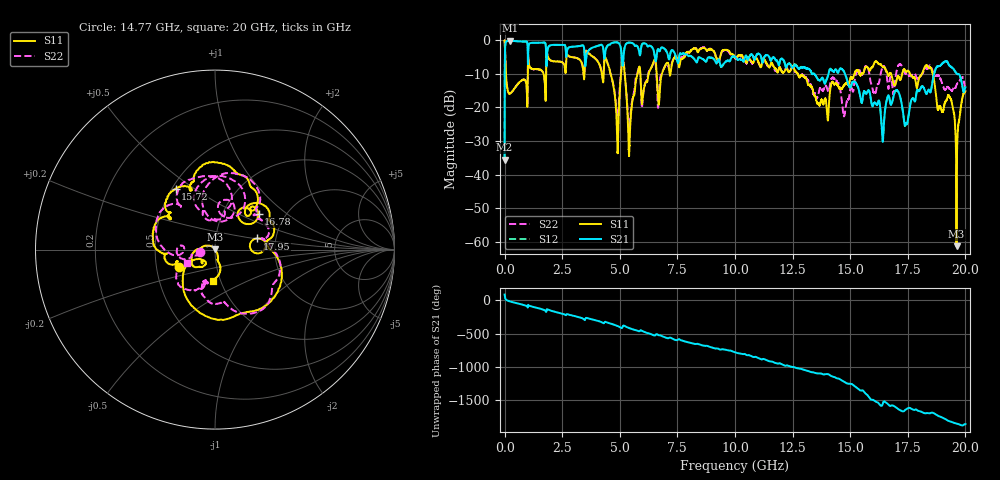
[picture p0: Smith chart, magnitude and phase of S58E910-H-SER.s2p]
!{S58E910}
!Johanson Technology Inc.
!www.johansontechnology.com
!Test Board Conditions:
!Substrate Type  RO4350B
!Substrate Thickness  60 mil
!Substrate Dk  3.66
!TL Type: GCPW
!TL Trace Width  115 mil
!TL Gap  52 mil
!Electrode orientation  Horizontal
!DUT TOPOLOGY	SERIES
!Mounting Pad LxW  55x428 mil
! Created Wed Apr 14 12:04:52 2021
# mhz S ma R 50
! 2 Port Network Data from SP1.SP block
! freq  magS11  angS11  magS21  angS21  magS12  angS12  magS22  angS22
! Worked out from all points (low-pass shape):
!   20001 points, 300 kHz to 20 GHz, reference 50 ohm
!   highest |S21| = -0.13 dB at 227.3 MHz (marker M1); lowest = -35.6 dB at 300 kHz (marker M2)
!   |S21| within 3 dB of the highest: 17.58 MHz to 1.006 GHz (988.3 MHz wide, 193 % of centre); 1.857 GHz to 2.657 GHz (800.7 MHz wide, 35.5 % of centre)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
!   lowest |S11| = -61.4 dB at 19.61 GHz (marker M3), VSWR 1.00, Z = 50 + j0.0846 ohm
!   |S11| at or under -10 dB: 57.03 MHz to 1.006 GHz (949.2 MHz wide, 179 % of centre); 12.73 GHz to 15.19 GHz (2.46 GHz wide, 17.6 % of centre); 18.58 GHz to end of sweep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
!   |S22| runs from -26.4 to 0.0 dB; largest |S21 - S12| = 0.016
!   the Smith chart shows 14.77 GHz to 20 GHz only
!   S11 on the Smith chart (normalised r, x): 14.77 GHz: 0.66, -0.13; 15.72 GHz: 0.52, +0.42; 16.78 GHz: 1.47, +0.65; 17.95 GHz: 1.59, +0.21; 20 GHz: 0.92, -0.33
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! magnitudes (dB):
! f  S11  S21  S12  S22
! 300 kHz  0.0  -35.6  -35.5  0.0
! 103.3 MHz  -13.7  -0.2  -0.2  -13.7
! 227.3 MHz  -15.9  -0.1  -0.1  -15.8
! 3.334 GHz  -6.5  -1.6  -1.6  -6.4
! 4.431 GHz  -6.1  -2.0  -1.9  -6.0
! 4.888 GHz  -29.1  -0.6  -0.6  -22.6
! 5.144 GHz  -6.3  -6.3  -6.3  -5.5
! 5.416 GHz  -32.3  -0.7  -0.7  -25.8
! 5.796 GHz  -9.3  -2.2  -2.2  -8.9
! 6.667 GHz  -18.1  -2.6  -2.6  -19.8
! 10 GHz  -5.2  -4.8  -4.8  -5.3
! 13.33 GHz  -13.9  -9.9  -9.9  -14.2
! 14.77 GHz  -13.1  -9.9  -9.9  -21.7
! 15.72 GHz  -7.9  -15.8  -15.8  -7.7
! 16.41 GHz  -7.9  -30.1  -29.9  -7.9
! 16.67 GHz  -10.6  -16.4  -16.4  -14.3
! 16.78 GHz  -10.1  -19.1  -19.2  -11.1
! 17.43 GHz  -9.4  -24.8  -24.8  -10.0
! 17.95 GHz  -12.3  -15.1  -14.9  -11.2
! 19.32 GHz  -17.0  -7.7  -7.6  -14.5
! 19.61 GHz  -61.4  -9.9  -9.8  -13.3
! 20 GHz  -15.2  -14.0  -13.9  -15.1
